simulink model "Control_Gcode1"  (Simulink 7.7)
settings: Solver=FixedStepDiscrete  SolverMode=SingleTasking  StartTime=0  StopTime=inf  FixedStep=dt  RelTol=1e-3  SampleTimeConstraint=Specified
InitFcn:
  | % Sampling Times %
  | dt0=0.001; dt1=0.01; samples=10;
undefined symbols (not defined in the file or in its folder): DiscIntNeverNeededParam, Volts
libraries: simulink_extras x4, speedgoatlib_IO311 x3, xpclib x3, simulink x3, speedgoatlib x2

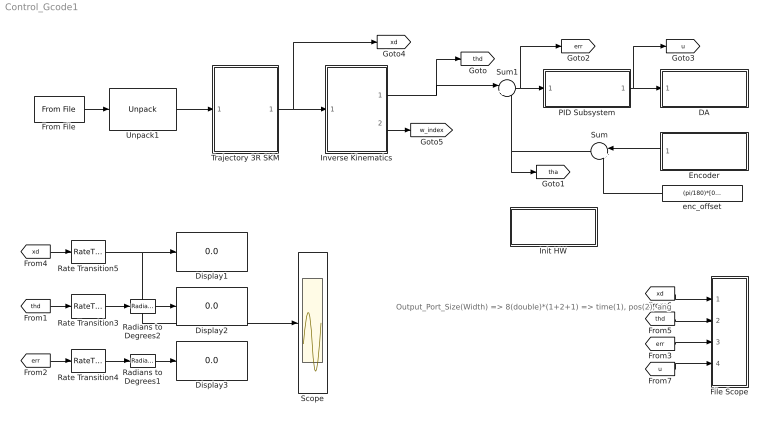
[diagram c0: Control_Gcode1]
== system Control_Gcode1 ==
  note: Output_Port_Size(Width) => 8(double)*(1+2+1) => time(1), pos(2), ang
  DA : Subsystem  TreatAsAtomicUnit=on
  Display1 : Display
  Display2 : Display
  Display3 : Display
  Encoder : Subsystem  TreatAsAtomicUnit=on
  File Scope : Subsystem
  From File : xpclib/Misc./From File  filename='skm2.dat'  dataSize=32  bufSize=4000  readSize=1024  EOFOption=Hold last output  sampTime=dt0
  Init HW : Subsystem  TreatAsAtomicUnit=on
  Inverse Kinematics : Stateflow chart  TreatAsAtomicUnit=on
  PID Subsystem : Subsystem  TreatAsAtomicUnit=on
  Radians to Degrees1 : simulink_extras/Transformations/Radians to Degrees  SystemSampleTime=-1
  Radians to Degrees2 : simulink_extras/Transformations/Radians to Degrees  SystemSampleTime=-1
  Rate Transition3 : RateTransition  OutPortSampleTime=dt1
  Rate Transition4 : RateTransition  OutPortSampleTime=dt1
  Rate Transition5 : RateTransition  OutPortSampleTime=dt1
  Scope : Scope
  Sum : Sum  Inputs=|++
  Sum1 : Sum  Inputs=|+-
  Trajectory 3R SKM : Stateflow chart  TreatAsAtomicUnit=on
  Unpack1 : xpclib/UDP/Unpack  dimensions={[4]}  datatypes={'double'}  byteAlign=1
  enc_offset : Constant  Value=(pi/180)*[0,90,0]'
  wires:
  [thd] -> Rate Transition3/1
  [err] -> Rate Transition4/1
  [xd] -> Rate Transition5/1
  Rate Transition5/1 -> Display1/1, Scope/1
  Rate Transition3/1 -> Radians to Degrees2/1
  Rate Transition4/1 -> Radians to Degrees1/1
  Radians to Degrees2/1 -> Display2/1
  Radians to Degrees1/1 -> Display3/1
  [xd] -> File Scope/1(xd)
  [thd] -> File Scope/2(thd)
  [err] -> File Scope/3(err)
  [u] -> File Scope/4(u)
  From File/1 -> Unpack1/1
  Trajectory 3R SKM/1(xd) -> Inverse Kinematics/1(xd), [xd]
  Unpack1/1 -> Trajectory 3R SKM/1(traj)
  Sum1/1 -> PID Subsystem/1(In1), [err]
  PID Subsystem/1(Out1) -> [u], DA/1(In1)
  Encoder/1(Out1) -> Sum/1
  enc_offset/1 -> Sum/2
  Sum/1 -> Sum1/2, [tha]
  Inverse Kinematics/1(thd) -> Sum1/1, [thd]
  Inverse Kinematics/2(w_index) -> [w_index]

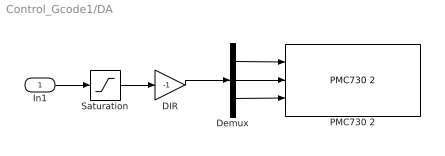
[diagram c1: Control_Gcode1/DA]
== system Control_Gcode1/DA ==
  In1 : Inport
  DIR : Gain  Gain=-1
  Demux : Demux  Outputs=3
  PMC730 2 : speedgoatlib/IO101/PMC730 2  id=1  channel=[1,2,3]  reset=[1,1,1]  initValue=[0,0,0]  ts=dt0  pciSlot=-1
  Saturation : Saturate  UpperLimit=10  LowerLimit=-10
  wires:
  In1/1 -> Saturation/1
  Saturation/1 -> DIR/1
  DIR/1 -> Demux/1
  Demux/1 -> PMC730 2/1
  Demux/2 -> PMC730 2/2
  Demux/3 -> PMC730 2/3

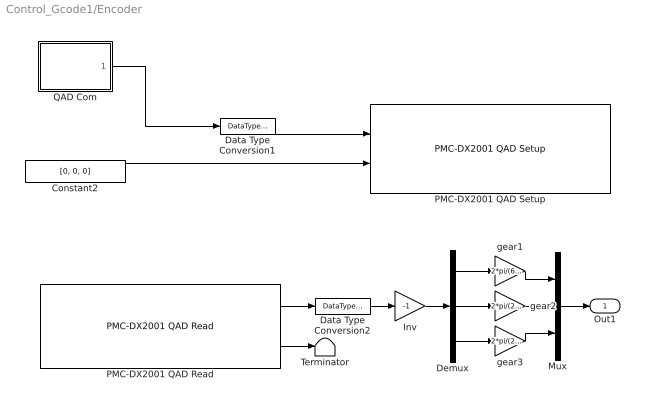
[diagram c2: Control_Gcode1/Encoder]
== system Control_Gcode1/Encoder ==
  Constant2 : Constant  Value=[0, 0, 0]  OutDataTypeStr=Inherit: Inherit via back propagation
  Data Type Conversion1 : DataTypeConversion  OutDataTypeStr=uint8
  Data Type Conversion2 : DataTypeConversion  OutDataTypeStr=double
  Demux : Demux  Outputs=3
  Inv : Gain  Gain=-1
  Mux : Mux  Inputs=3
  PMC-DX2001 QAD Read : speedgoatlib_IO311/PMC-DX2001 QAD Read  id=1  chan=[1, 2, 3]  pciSlot=-1  ts=dt0
  PMC-DX2001 QAD Setup : speedgoatlib_IO311/PMC-DX2001 QAD Setup  id=1  chan=Channel 3 setup  steps1=2000  steps2=2000  steps3=2000  quadrature1=4x  quadrature2=4x  quadrature3=4x  index1=Ignore index input  index2=Ignore index input  index3=Ignore index input  special1=Disabled (cycling counter)  special2=Disabled (cycling counter)  special3=Disabled (cycling counter)  debounce=0  pciSlot=-1  ts=dt0
  QAD Com : Stateflow chart  TreatAsAtomicUnit=on
  Terminator : Terminator
  gear1 : Gain  Gain=2*pi/(66*2000)
  gear2 : Gain  Gain=2*pi/(23*2000)
  gear3 : Gain  Gain=2*pi/(23*2000)
  Out1 : Outport
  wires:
  Constant2/1 -> PMC-DX2001 QAD Setup/2
  PMC-DX2001 QAD Read/2 -> Terminator/1
  PMC-DX2001 QAD Read/1 -> Data Type Conversion2/1
  QAD Com/1(y) -> Data Type Conversion1/1
  Data Type Conversion1/1 -> PMC-DX2001 QAD Setup/1
  Data Type Conversion2/1 -> Inv/1
  Mux/1 -> Out1/1
  Demux/1 -> gear1/1
  gear1/1 -> Mux/1
  Demux/2 -> gear2/1
  gear2/1 -> Mux/2
  Inv/1 -> Demux/1
  Demux/3 -> gear3/1
  gear3/1 -> Mux/3

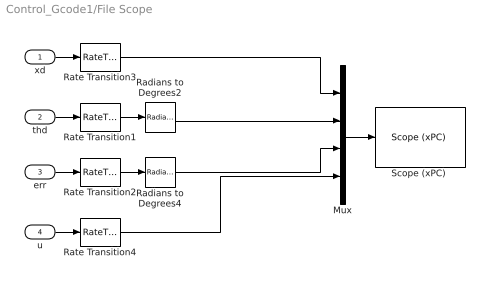
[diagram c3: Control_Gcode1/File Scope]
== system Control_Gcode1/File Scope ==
  xd : Inport
  thd : Inport  Port=2
  err : Inport  Port=3
  u : Inport  Port=4
  Mux : Mux
  Radians to Degrees2 : simulink_extras/Transformations/Radians to Degrees  SystemSampleTime=-1
  Radians to Degrees4 : simulink_extras/Transformations/Radians to Degrees  SystemSampleTime=-1
  Rate Transition{1..4} (4 alike) : RateTransition  OutPortSampleTime=dt1
  "Scope (xPC) " : xpclib/Misc./Scope (xPC)   SystemSampleTime=-1  scopeno=2  scopetype=File  autostart=on  viewmode=Graphical redraw  formatstr='%15.6f'  grid=on  ylimits=[0,0]  nosamples=100  noprepostsamples=0  interleave=1  triggermode=FreeRun  triggersignal=1  triggerlevel=0.0  triggerslope=Either  triggerscope=1  triggersample=0  filename=step3.dat  mode=Lazy  writesize=512  autorestart=on  dynamicfilemode=off  maxwritefilesize=512*1024^2
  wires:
  Radians to Degrees2/1 -> Mux/2
  Radians to Degrees4/1 -> Mux/3
  Rate Transition1/1 -> Radians to Degrees2/1
  Rate Transition2/1 -> Radians to Degrees4/1
  thd/1 -> Rate Transition1/1
  err/1 -> Rate Transition2/1
  Rate Transition3/1 -> Mux/1
  xd/1 -> Rate Transition3/1
  u/1 -> Rate Transition4/1
  Mux/1 -> "Scope (xPC) "/1
  Rate Transition4/1 -> Mux/4

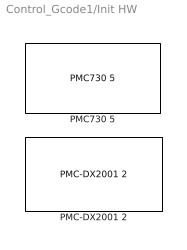
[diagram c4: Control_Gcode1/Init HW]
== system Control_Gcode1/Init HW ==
  PMC-DX2001 2 : speedgoatlib_IO311/PMC-DX2001 2  id=1  fpga1=IO311_3PWM_3CAP_3QAD_INT.fpga  fpga2=PWM_Triangle_DX501.fpga  fpga3=PWM_Triangle_DX501.fpga  fpga4=PWM_Triangle_DX501.fpga  fpga5=PWM_Triangle_DX501.fpga  fpga6=PWM_Triangle_DX501.fpga  fpga7=PWM_Triangle_DX501.fpga  fpga8=PWM_Triangle_DX501.fpga  fpga9=PWM_Triangle_DX501.fpga  fpga10=PWM_Triangle_DX501.fpga  group=Module setup  pciSlot=-1  lowerDirection=[ones(1,5), zeros(1, 7), ones(1, 1), ones(1, 3)]  lowerReset=[1]  lowerValue=[0]  upperDirection=[ones(1, 8), zeros(1, 8)]  upperReset=[1]  upperValue=[0]
  PMC730 5 : speedgoatlib/IO101/PMC730 5  id=1  group=Analog output setup  pciSlot=-1  adStartChannel=1  adNumChannel=1  adCoupling=Single-ended  adRange=-10 .. 10 Volts  adAcqMode=Standard  daChannel=[1,2, 3]  daReset=[1,1, 1]  daInitValue=[0,0,0]  diChannel=[1]  diDebounce=[0]  doChannel=[1]  doReset=[1]  doInitValue=[0]

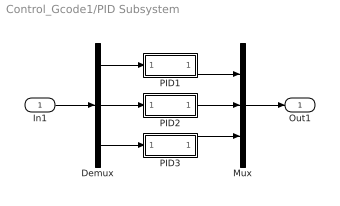
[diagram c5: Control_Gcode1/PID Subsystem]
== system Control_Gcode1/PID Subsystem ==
  In1 : Inport
  Demux : Demux  Outputs=3
  Mux : Mux  Inputs=3
  PID1 : Subsystem
  PID2 : Subsystem
  PID3 : Subsystem
  Out1 : Outport
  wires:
  In1/1 -> Demux/1
  Demux/1 -> PID1/1(In1)
  PID1/1(Out1) -> Mux/1
  Demux/2 -> PID2/1(In1)
  PID2/1(Out1) -> Mux/2
  Mux/1 -> Out1/1
  Demux/3 -> PID3/1(In1)
  PID3/1(Out1) -> Mux/3

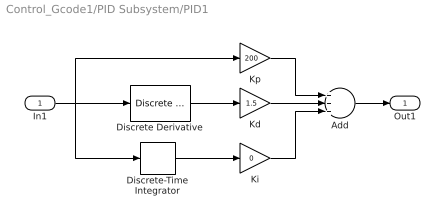
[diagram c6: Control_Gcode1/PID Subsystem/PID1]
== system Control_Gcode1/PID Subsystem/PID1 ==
  In1 : Inport
  Add : Sum  Inputs=+++
  Discrete Derivative : simulink/Discrete/Discrete Derivative  SystemSampleTime=-1  gainval=1.0  ICPrevScaledInput=0.0  OutMin=[]  OutMax=[]  OutDataType=fixdt(1, 16)  OutScaling=2^-10  DoSatur=off
  Discrete-Time Integrator : DiscreteIntegrator  SampleTime=dt0  ICPrevOutput=DiscIntNeverNeededParam  ICPrevScaledInput=DiscIntNeverNeededParam
  Kd : Gain  Gain=1.5
  Ki : Gain  Gain=0
  Kp : Gain  Gain=200
  Out1 : Outport
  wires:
  Discrete-Time Integrator/1 -> Ki/1
  Kp/1 -> Add/1
  Kd/1 -> Add/2
  Ki/1 -> Add/3
  Discrete Derivative/1 -> Kd/1
  Add/1 -> Out1/1
  In1/1 -> Kp/1, Discrete Derivative/1, Discrete-Time Integrator/1

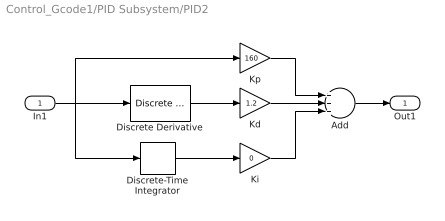
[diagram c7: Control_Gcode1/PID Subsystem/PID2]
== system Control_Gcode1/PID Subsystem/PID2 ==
  In1 : Inport
  Add : Sum  Inputs=+++
  Discrete Derivative : simulink/Discrete/Discrete Derivative  SystemSampleTime=-1  gainval=1.0  ICPrevScaledInput=0.0  OutMin=[]  OutMax=[]  OutDataType=fixdt(1, 16)  OutScaling=2^-10  DoSatur=off
  Discrete-Time Integrator : DiscreteIntegrator  SampleTime=dt0  ICPrevOutput=DiscIntNeverNeededParam  ICPrevScaledInput=DiscIntNeverNeededParam
  Kd : Gain  Gain=1.2
  Ki : Gain  Gain=0
  Kp : Gain  Gain=160
  Out1 : Outport
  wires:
  Discrete-Time Integrator/1 -> Ki/1
  Kp/1 -> Add/1
  Kd/1 -> Add/2
  Ki/1 -> Add/3
  Discrete Derivative/1 -> Kd/1
  Add/1 -> Out1/1
  In1/1 -> Kp/1, Discrete Derivative/1, Discrete-Time Integrator/1

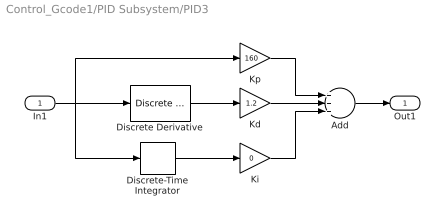
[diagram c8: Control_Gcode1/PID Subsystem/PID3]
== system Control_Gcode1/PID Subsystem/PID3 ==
  In1 : Inport
  Add : Sum  Inputs=+++
  Discrete Derivative : simulink/Discrete/Discrete Derivative  SystemSampleTime=-1  gainval=1.0  ICPrevScaledInput=0.0  OutMin=[]  OutMax=[]  OutDataType=fixdt(1, 16)  OutScaling=2^-10  DoSatur=off
  Discrete-Time Integrator : DiscreteIntegrator  SampleTime=dt0  ICPrevOutput=DiscIntNeverNeededParam  ICPrevScaledInput=DiscIntNeverNeededParam
  Kd : Gain  Gain=1.2
  Ki : Gain  Gain=0
  Kp : Gain  Gain=160
  Out1 : Outport
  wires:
  Discrete-Time Integrator/1 -> Ki/1
  Kp/1 -> Add/1
  Kd/1 -> Add/2
  Ki/1 -> Add/3
  Discrete Derivative/1 -> Kd/1
  Add/1 -> Out1/1
  In1/1 -> Kp/1, Discrete Derivative/1, Discrete-Time Integrator/1

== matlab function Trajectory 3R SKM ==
function xd = fcn(traj)

a1=100; a2=70; a3=50;

x0=[a1,a2+a3, pi/2]';
xd=x0+traj(2:4,1);

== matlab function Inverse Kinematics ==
function [thd,w_index]  = fcn(xd)

persistent index thd_p

% Initializing Variables %
if isempty(index), index=0; end
if isempty(thd_p), thd_p=(pi/180)*[0,90,0]'; end

w_index=1;  % In workspace %
a1=100; a2=70; a3=50;

qx=xd(1,1); qy=xd(2,1); phi=xd(3,1);

% (1) Calculate th2 %
px=qx-a3*cos(phi); py=qy-a3*sin(phi);
kapha=(px^2+py^2-a1^2-a2^2)/(2*a1*a2);
if abs(kapha)>1
    w_index=-1;  % Out of Workspace %
    kapha=1;
end
th2=+acos(kapha); % Elbow Down %
%th2=-acos(kapha); % Elbow Up %
 
% (2) Calculate th1 %
delta=a1^2+a2^2+2*a1*a2*cos(th2);
cth1=(px*(a1+a2*cos(th2))+py*a2*sin(th2))/delta;
sth1=(-px*a2*sin(th2)+py*(a1+a2*cos(th2)))/delta;
th1=atan2(sth1, cth1);
if th1<0, th1=th1+2*pi; end % 0<th<360 %

% (3) Calcuate th3 %
th3=phi-(th1+th2);

% (3) Check Joint Limits %
if th1<0 || th1>pi, w_index=-1; end
if th2<pi/6 || th2>5*pi/6, w_index=-1; end

% Result %
if w_index==1
    thd=[th1, th2, th3]';
else
    thd=thd_p;
end

% Save the current value %
thd_p=thd;

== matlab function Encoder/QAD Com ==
function y = fcn()

persistent index

if isempty(index), index=0; end

if index==0
    y=[1,1,1];      %  Reset %
else
    y = [0,0,0];
end

index=index+1;
